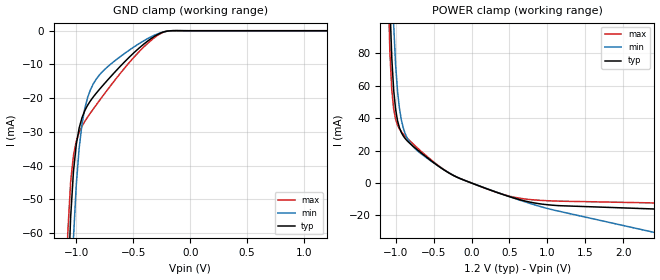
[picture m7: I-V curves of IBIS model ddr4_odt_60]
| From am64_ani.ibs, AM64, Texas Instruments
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|   Model ddr4_odt_60
[Model] ddr4_odt_60
Model_type Input
Polarity   Non-Inverting
Enable   Active-High
Vinl =  0.700V
Vinh =  0.900V
C_comp   2.403pF   2.372pF   2.539pF
[Model Spec]
Vinh   0.900V   0.820V   0.980V
Vinl   0.700V   0.620V   0.780V
[Temperature Range]   25.000   0.125k   -40.000
[Voltage Range]   1.200V   1.140V   1.260V
[C Comp Corner]
C_comp   2.403pF   2.372pF   2.539pF
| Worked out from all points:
|   GND clamp passes 1 mA (typ) near -0.28 V on its own axis
|   POWER clamp passes 1 mA (typ) near -0.06 V on its own axis
[GND_clamp]
|Voltage   I(typ)   I(min)   I(max)
-1.2V     -388.2mA   -434.9mA   -364.4mA
-1.075V   -77.92mA   -117.2mA   -60.12mA
-1.05V    -55.4mA    -84.81mA   -44.9mA
-1.025V   -41.74mA   -61.56mA   -37mA
-1V       -33.68mA   -45.54mA   -32.73mA
-975mV    -28.85mA   -34.82mA   -30.14mA
-950mV    -25.78mA   -27.71mA   -28.32mA
-900mV    -22.05mA   -19.72mA   -25.56mA
-800mV    -17.51mA   -13.23mA   -20.84mA
-575mV    -9.193mA   -6.717mA   -11.03mA
-200mV    -109.4uA   -106.7uA   -117.5uA
1.2V      0A         0A         0A
[POWER_clamp]
|Voltage   I(typ)   I(min)   I(max)
-1.2V     598.1mA    737mA      625.7mA
-1.1V     161.3mA    252.8mA    124.1mA
-1.075V   109.8mA    183.6mA    80.44mA
-1.05V    76.96mA    132.9mA    57.36mA
-1.025V   57.16mA    97.27mA    45.6mA
-1V       45.49mA    73.11mA    39.37mA
-975mV    38.51mA    56.99mA    35.74mA
-925mV    31.21mA    39.07mA    31.63mA
-825mV    24.98mA    25.79mA    26.59mA
-325mV    6.978mA    7.081mA    7.071mA
650mV     -10.45mA   -10.77mA   -9.48mA
2.4V      -15.99mA   -30.37mA   -12.27mA
